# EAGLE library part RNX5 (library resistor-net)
RESISTOR NETWORK
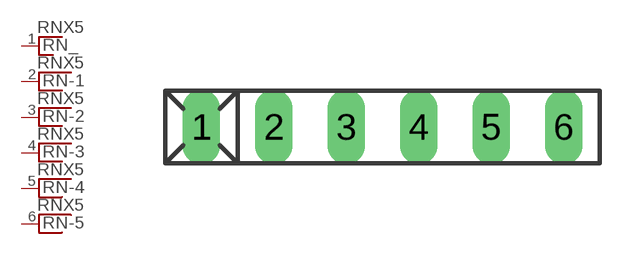
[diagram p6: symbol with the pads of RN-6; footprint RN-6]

Designator prefix RN; gates _=RN_1 -1=RNX -2=RNX -3=RNX -4=RNX -5=RNX

## RNX5 (OC_FARNELL: unknown; OC_NEWARK: unknown)  [RN-6]
1  _:1  pas
2  -1:1  pas
3  -2:1  pas
4  -3:1  pas
5  -4:1  pas
6  -5:1  pas

## Footprint RN-6 (pad centres in mm)
RESISTOR NETWORK
drill 0.813 long: 1 -6.35,0; 2 -3.81,0; 3 -1.27,0; 4 1.27,0; 5 3.81,0; 6 6.35,0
